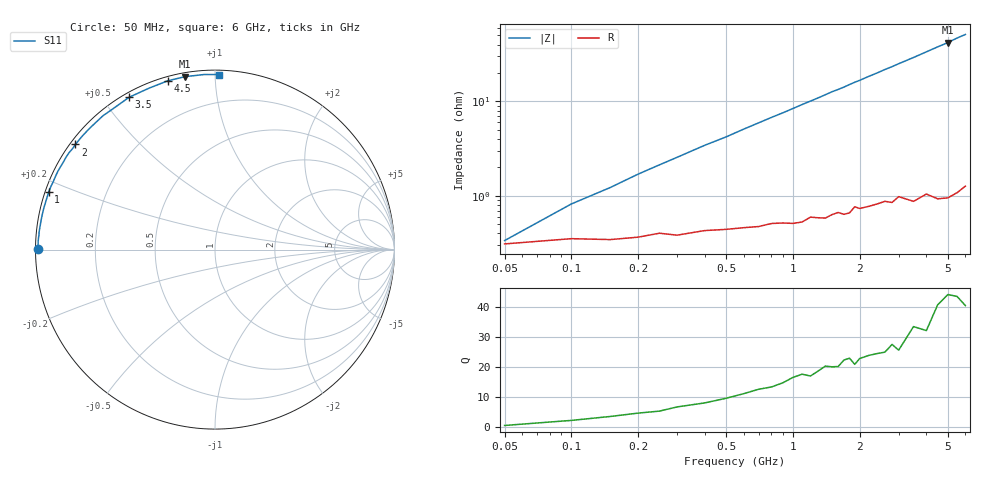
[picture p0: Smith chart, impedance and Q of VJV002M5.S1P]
! Infineon Technologies  Discrete & RF Semiconductors
! BB 914
! Si Tuning Diode in SOT23
! VR =
! S-Parameters:  July  1999
# GHz  S  MA  R  50
!  f  S11
! GHz  MAG  ANG
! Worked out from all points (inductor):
!   34 points, 50 MHz to 6 GHz, reference 50 ohm
!   read as one part to ground: L = 1.32 nH near 150 MHz
!   highest Q = 43.5 at 5 GHz (marker M1), where L = 1.34 nH
!   S11 on the Smith chart (normalised r, x): 50 MHz: 0.01, +0.00; 1 GHz: 0.01, +0.17; 2 GHz: 0.01, +0.33; 3.5 GHz: 0.02, +0.58; 4.5 GHz: 0.02, +0.76; 6 GHz: 0.03, +1.02
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0.05  0.9877 179.7
0.1  0.986 178.3
0.3  0.9848 174.2
0.4  0.9831 172.2
0.5  0.9826 170.4
0.6  0.9819 168.4
0.8  0.9802 164.6
1  0.9803 160.9
1.1  0.9798 159.0
1.3  0.9779 155.4
1.4  0.9782 153.5
1.5  0.9765 151.6
1.6  0.9754 150.0
1.7  0.9767 148.3
1.8  0.9761 146.4
1.9  0.9725 144.6
2  0.9739 143.0
2.2  0.9731 139.5
2.4  0.9721 136.3
2.6  0.971 132.9
2.8  0.9724 129.9
3  0.9691 126.7
3.5  0.9742 119.4
4  0.9716 112.3
4.5  0.9766 105.7
5  0.9779 99.9
5.5  0.9773 93.6
6  0.9756 88.6
